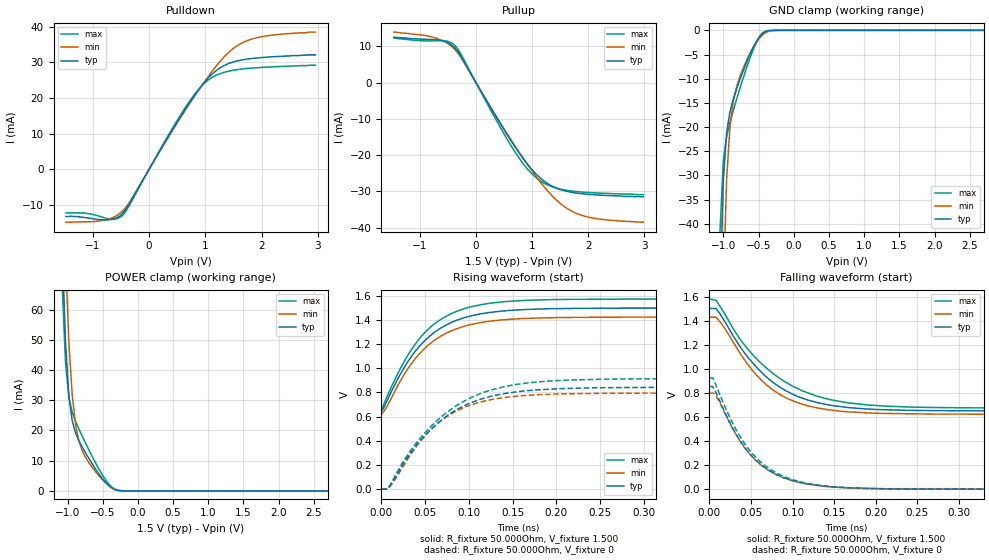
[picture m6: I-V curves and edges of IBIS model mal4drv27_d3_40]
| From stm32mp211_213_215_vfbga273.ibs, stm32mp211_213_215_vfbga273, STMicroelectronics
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[Model] mal4drv27_d3_40
Model_type   I/O
Polarity   Non-Inverting
Enable   Active-High
C_comp   1.653pF   1.649pF   1.658pF
C_comp_pullup   821.240fF   815.174fF   828.427fF
C_comp_pulldown 737.945fF   733.914fF   744.436fF
Vinh = 885.000mV
Vinl = 615.000mV
Vmeas = 750.000mV
Vref = 750.000mV
Rref = 50Ohms
Cref = 0pF
[Model Spec]
Vinh   885.000mV   848.000mV   923.000mV
Vinl   615.000mV   578.000mV   653.000mV
Vmeas   750.000mV   713.000mV   788.000mV
Vref   750.000mV   713.000mV   788.000mV
D_overshoot_ampl_h 0.4 NA   NA
D_overshoot_ampl_l 0.4 NA   NA
D_overshoot_area_l 100.000m NA   NA
D_overshoot_area_h 100.000m NA   NA
[Receiver Thresholds]
Vth = 750.000mV
Vth_min = 713.000mV
Vth_max = 788.000mV
Vinh_ac = 135.000mV
Vinh_dc = 100.000mV
Vinl_ac = -135.000mV
Vinl_dc = -100.000mV
Tslew_ac = 5.000ns
Threshold_sensitivity = 0.5
Reference_supply Pullup_ref
[Temperature Range]   25.000   125.000   -40.000
[Voltage Range]   1.500V   1.425V   1.575V
[GND Clamp Reference]   0.00V   0.00V   0.00V
[C Comp Corner]
| variable   typ   min   max
C_comp 1.658pF   1.653pF   1.649pF
C_comp_pullup 821.240fF   828.427fF   815.174fF
C_comp_pulldown 733.914fF   744.436fF   737.945fF
[Pulldown Reference]   0.00V   0.00V   0.00V
[POWER Clamp Reference]   1.500V   1.425V   1.575V
[Pullup Reference]   1.500V   1.425V   1.575V
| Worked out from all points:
|   slope of the pulldown table from 0 to 0.225 V, typ, clamps not added: 36.9 ohm
|   slope of the pullup table from 0 to 0.225 V, typ, clamps not added: 37.6 ohm
|   GND clamp passes 1 mA (typ) near -0.47 V on its own axis
|   POWER clamp passes 1 mA (typ) near -0.37 V on its own axis
|   rising waveform, R_fixture 50.000Ohm, V_fixture 1.500: 20-80 % time 54.8ps typ, 53.9ps min, 53.7ps max; typ from 0.643 V to 1.5 V
|   rising waveform, R_fixture 50.000Ohm, V_fixture 0: 20-80 % time 68.6ps typ, 60.7ps min, 74ps max; typ from -0.003 V to 0.842 V
|   falling waveform, R_fixture 50.000Ohm, V_fixture 1.500: 20-80 % time 67.6ps typ, 60.7ps min, 77.1ps max; typ from 1.5 V to 0.65 V
|   falling waveform, R_fixture 50.000Ohm, V_fixture 0: 20-80 % time 52.9ps typ, 52.2ps min, 53.6ps max; typ from 0.852 V to 0 V
[GND Clamp]
-1.48V    -1.356A    -1.372A    -1.368A
-1.05V    -57.52mA   -98.82mA   -41.99mA
-1.002V   -31.12mA   -53.93mA   -27.05mA
-954.6mV  -21.13mA   -30.8mA    -21.99mA
-906.8mV  -16.83mA   -19.93mA   -19.06mA
-859.1mV  -14.2mA    -14.62mA   -16.56mA
-763.6mV  -10.09mA   -9.457mA   -11.91mA
-668.2mV  -6.482mA   -6.16mA    -7.611mA
-525mV    -2.097mA   -2.366mA   -2.333mA
-429.5mV  -449.8uA   -771.1uA   -394uA
-238.6mV  -1.709uA   -14.74uA   -370nA
2.959V    53.06nA    707.1nA    76.78nA
[Power Clamp]
-1.459V   570.2mA    591.8mA    567.2mA
-1.077V   80.71mA    114.2mA    68.27mA
-1.03V    49.21mA    76.71mA    42.66mA
-981.8mV  31.4mA     49.26mA    30.9mA
-934.1mV  23.16mA    31.72mA    25.95mA
-886.4mV  19.16mA    21.79mA    22.98mA
-838.6mV  16.6mA     16.39mA    20.46mA
-743.2mV  12.52mA    11.03mA    15.74mA
-647.7mV  8.857mA    7.696mA    11.27mA
-361.4mV  773.2uA    986uA      1.034mA
-218.2mV  12.39uA    63.5uA     9.952uA
2.98V     -55.08nA   -1.144uA   -55.82nA
[Pulldown]
-1.48V    -13.3mA    -14.9mA    -12.3mA
-1.145V   -13.6mA    -14.8mA    -12.3mA
-763.6mV  -14.27mA   -14.2mA    -13.82mA
-477.3mV  -12.52mA   -11.82mA   -13.04mA
-334.1mV  -9.248mA   -8.873mA   -9.642mA
286.4mV   7.739mA    7.529mA    8.025mA
668.2mV   17.44mA    17.17mA    17.88mA
906.8mV   22.84mA    22.83mA    22.91mA
1.145V    27.06mA    28mA       25.99mA
1.48V     30.02mA    33.66mA    27.72mA
1.766V    30.96mA    36.22mA    28.31mA
2.959V    32.1mA     38.5mA     29.2mA
[Pullup]
-1.459V   12.5mA     13.9mA     12.26mA
-743.2mV  11.82mA    12.39mA    11.49mA
-504.6mV  11.02mA    10.78mA    11.37mA
-361.4mV  9.327mA    8.847mA    10.02mA
-265.9mV  7.185mA    6.86mA     7.818mA
688.6mV   -17.57mA   -17.29mA   -18.96mA
927.3mV   -22.7mA    -22.8mA    -24.01mA
1.166V    -26.6mA    -27.81mA   -27.31mA
1.5V      -29.49mA   -33.31mA   -29.37mA
1.834V    -30.57mA   -36.35mA   -30.12mA
2.264V    -31.08mA   -37.77mA   -30.52mA
2.98V     -31.5mA    -38.5mA    -30.9mA
[Ramp]
R_load=50.000Ohm
dV/dt_r   507.690mV/62.500ps  479.158mV/58.500ps  544.530mV/65.000ps
dV/dt_f   507.720mV/61.500ps  479.159mV/57.500ps  544.530mV/66.500ps
[Rising waveform]
R_fixture=50.000Ohm
V_fixture=1.500
V_fixture_min=1.425
V_fixture_max=1.575
0s        643.2mV    619.5mV    661.1mV
6ps       723.9mV    678.9mV    757.3mV
24ps      981.3mV    925.1mV    1.03V
36ps      1.116V     1.055V     1.174V
46ps      1.203V     1.14V      1.268V
72ps      1.352V     1.284V     1.425V
104ps     1.438V     1.366V     1.514V
143ps     1.478V     1.405V     1.555V
192ps     1.495V     1.42V      1.57V
469ps     1.5V       1.425V     1.575V
[Rising waveform]
R_fixture=50.000Ohm
V_fixture=0
0s        -3.299mV   -3.191mV   -1.775mV
7ps       -3.299mV   -3.191mV   -1.775mV
34ps      303.6mV    289.5mV    324.3mV
49ps      436.7mV    431.5mV    459.4mV
65ps      549mV      545.6mV    575.6mV
91ps      676.4mV    663.5mV    712.9mV
126ps     768.4mV    740.7mV    821.7mV
156ps     806.3mV    769.8mV    868mV
209ps     832.2mV    788.3mV    901.3mV
476ps     842.2mV    794.7mV    914.2mV
[Falling waveform]
R_fixture=50.000Ohm
V_fixture=1.500
V_fixture_min=1.425
V_fixture_max=1.575
0s        1.501V     1.428V     1.579V
8ps       1.501V     1.428V     1.569V
12ps      1.464V     1.398V     1.528V
42ps      1.134V     1.076V     1.199V
56ps      1.017V     953mV      1.088V
73ps      906.5mV    842.1mV    979.8mV
106ps     770.6mV    718.7mV    835.9mV
143ps     700.3mV    659.8mV    746.8mV
227ps     656.3mV    626.7mV    684.8mV
477ps     649.9mV    622.5mV    674.2mV
[Falling waveform]
R_fixture=50.000Ohm
V_fixture=0
0s        852.4mV    798mV      924.4mV
4ps       852.4mV    798mV      924.4mV
9ps       787.1mV    761.6mV    846.7mV
30ps      482.1mV    477.3mV    521.6mV
51ps      275.8mV    271.9mV    300.8mV
75ps      143mV      139.8mV    156.7mV
102ps     67.36mV    65.52mV    74.59mV
130ps     31.05mV    29.67mV    34.13mV
178ps     7.837mV    7.731mV    8.991mV
473ps     795.1nV    6.103uV    0V
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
